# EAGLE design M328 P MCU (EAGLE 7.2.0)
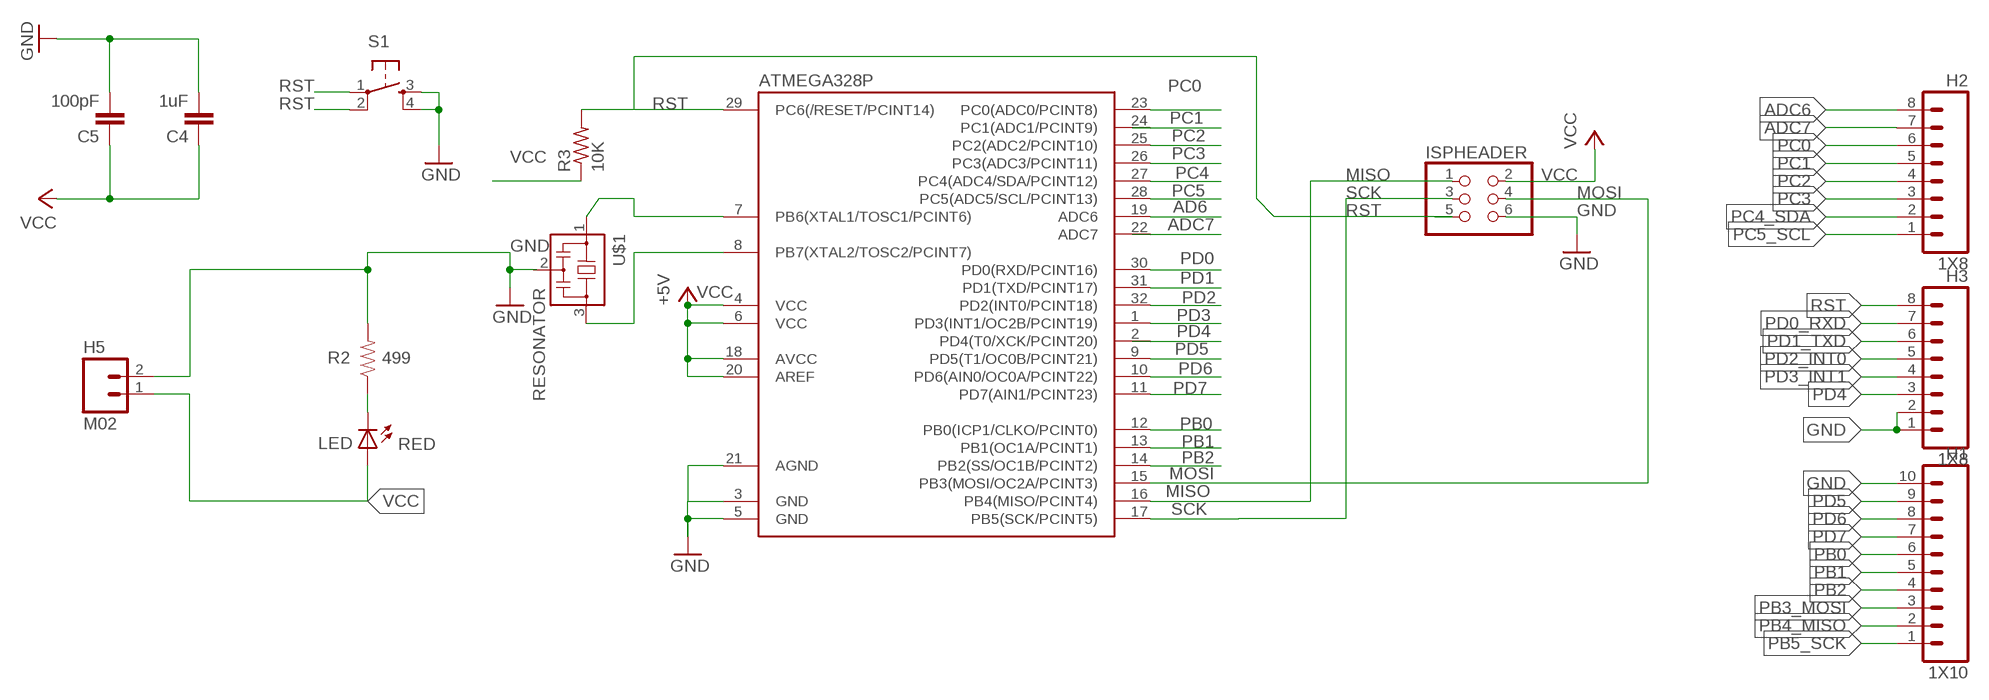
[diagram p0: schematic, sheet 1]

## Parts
ATMEGA328P  ATMEGA48/88/168-MU  [MLF32]
C4  1uF  CAP1206  [1206]
C5  100pF  CAP1206  [1206]
H1  1X10  M101X10_SMD_STRAIGHT_ALT  [1X10_SMD_STRAIGHT_ALT]
H2  1X8  M081X08_SMD_STRAIGHT_ALT  [1X08_SMD_STRAIGHT_ALT]
H3  1X8  M081X08_SMD_STRAIGHT_ALT  [1X08_SMD_STRAIGHT_ALT]
H5  M02  [1X02_SMD_FLAT_PADS]
ISPHEADER  PINHD-2X3-SMD  [2X03SMD]
LED  RED  LED1206  [1206]
R2  499  RESISTOR1206  [1206]
R3  10K  RESISTOR1206  [1206]
S1  6MM_SWITCH6MM_SWITCH  [6MM_SWITCH]
U$1  RESONATOR  [EFOBM]

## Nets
AD6: ATMEGA328P.19(ADC6)
ADC6: H2.8
ADC7: H2.7
GND: ATMEGA328P.3(GND) ATMEGA328P.5(GND) ATMEGA328P.21(AGND) C4.2 C5.2 H1.10 H3.1 H3.2 H5.2 ISPHEADER.6 R2.2 S1.3(S) S1.4(S1)
MISO: ATMEGA328P.16(PB4(MISO/PCINT4)) ISPHEADER.1
MOSI: ATMEGA328P.15(PB3(MOSI/OC2A/PCINT3)) ISPHEADER.4
N$1: ATMEGA328P.7(PB6(XTAL1/TOSC1/PCINT6)) U$1.1
N$2: ATMEGA328P.8(PB7(XTAL2/TOSC2/PCINT7)) U$1.3
N$26: LED.2(C) R2.1
PB0: ATMEGA328P.12(PB0(ICP1/CLKO/PCINT0)) H1.6
PB1: ATMEGA328P.13(PB1(OC1A/PCINT1)) H1.5
PB2: ATMEGA328P.14(PB2(SS/OC1B/PCINT2)) H1.4
PB3_MOSI: H1.3
PB4_MISO: H1.2
PB5_SCK: H1.1
PC0: ATMEGA328P.23(PC0(ADC0/PCINT8)) H2.6
PC1: H2.5
PC2: ATMEGA328P.25(PC2(ADC2/PCINT10)) H2.4
PC3: ATMEGA328P.26(PC3(ADC3/PCINT11)) H2.3
PC4: ATMEGA328P.27(PC4(ADC4/SDA/PCINT12))
PC4_SDA: H2.2
PC5: ATMEGA328P.28(PC5(ADC5/SCL/PCINT13))
PC5_SCL: H2.1
PD0: ATMEGA328P.30(PD0(RXD/PCINT16))
PD0_RXD: H3.7
PD1: ATMEGA328P.31(PD1(TXD/PCINT17))
PD1_TXD: H3.6
PD2: ATMEGA328P.32(PD2(INT0/PCINT18))
PD2_INT0: H3.5
PD3: ATMEGA328P.1(PD3(INT1/OC2B/PCINT19))
PD3_INT1: H3.4
PD4: H3.3
PD5: ATMEGA328P.9(PD5(T1/OC0B/PCINT21)) H1.9
PD6: ATMEGA328P.10(PD6(AIN0/OC0A/PCINT22)) H1.8
PD7: ATMEGA328P.11(PD7(AIN1/PCINT23)) H1.7
RST: ATMEGA328P.29(PC6(/RESET/PCINT14)) H3.8 ISPHEADER.5 R3.2 S1.1(P) S1.2(P1)
SCK: ATMEGA328P.17(PB5(SCK/PCINT5)) ISPHEADER.3
VCC: ATMEGA328P.4(VCC) ATMEGA328P.6(VCC) ATMEGA328P.18(AVCC) ATMEGA328P.20(AREF) C4.1 C5.1 H5.1 ISPHEADER.2 LED.1(A) R3.1 ; supply symbol labelled +5V
Unconnected: ATMEGA328P.2(PD4(T0/XCK/PCINT20)) ATMEGA328P.22(ADC7) ATMEGA328P.24(PC1(ADC1/PCINT9)) U$1.2

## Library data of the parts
ATMEGA328P = 01_atmega8:ATMEGA48/88/168
C4 C5 = 01_SparkFun:CAP: Capacitor
H1 = Working:M10
H2 H3 = Working:M08
H5 = Working:M02
ISPHEADER = 01_FAB_Hello:PINHD-2X3-SMD: PIN HEADER
LED = 01_FAB_Hello:LED
R2 = 01_SparkFun:RESISTOR: Resistor
R3 = 01_FAB_Hello:RESISTOR
S1 = 01_FAB_Hello:6MM_SWITCH: OMRON SWITCH
U$1 = fab-sp:RESONATOR

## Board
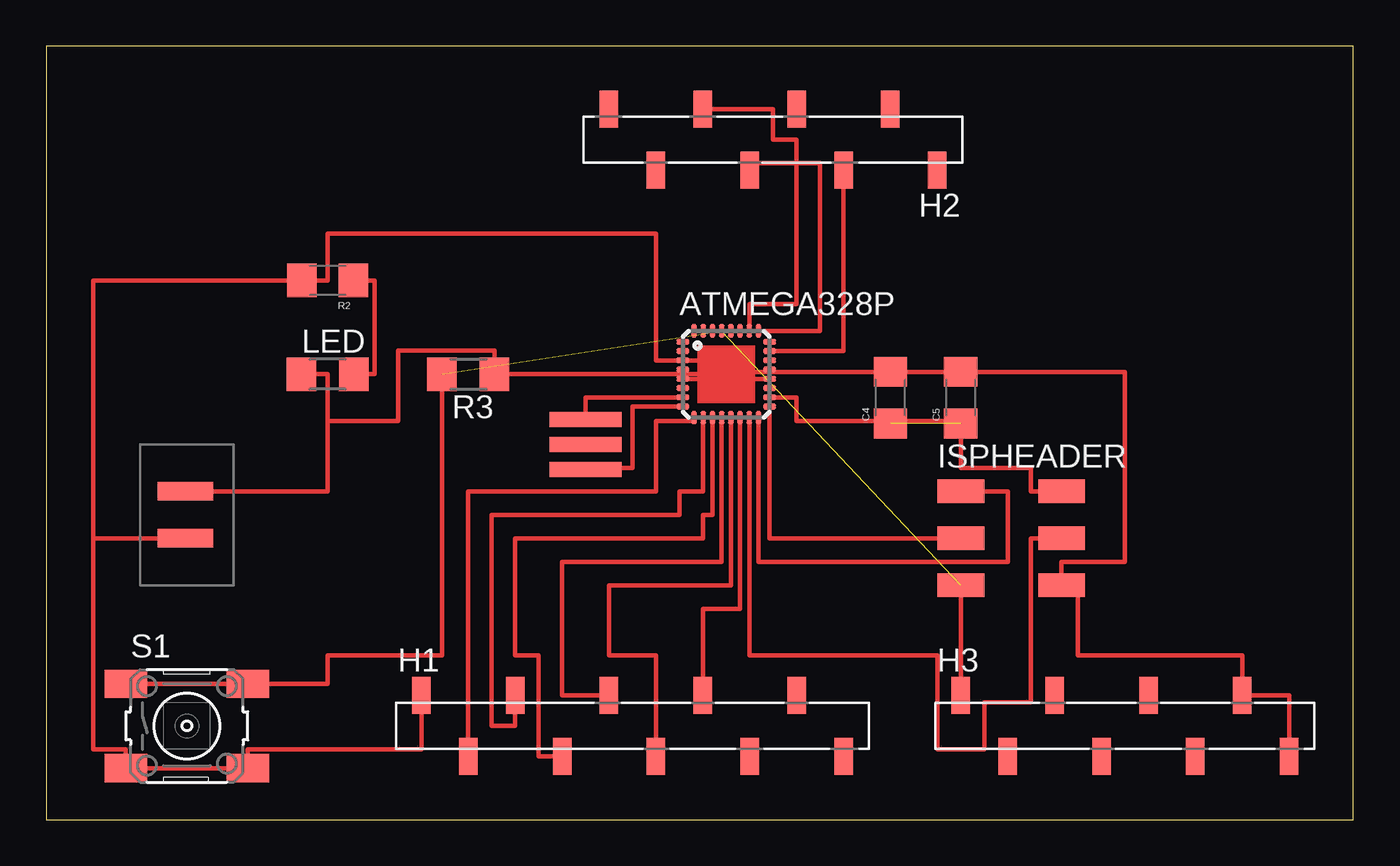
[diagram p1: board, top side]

Size 70.79 x 41.9 mm. Coordinates in mm from the lower left corner, seen from the top.
Outline: 0,0 70.79,0 70.79,41.9 0,41.9 0,0
Copper layers (1*16): Top 0.035mm / dielectric 1.5mm / Bottom 0.035mm
Design rules "default": minimum track width 10mil, minimum drill 24mil, track to track 8mil, track to pad 8mil, pad to pad 8mil, via to via 8mil, smd to smd 8mil, copper to edge 40mil, drill to drill 8mil, minimum pad ring 10mil, minimum via ring 8mil, stop-mask expansion 4mil, vias tented up to drill 0mil, thermal gap 10mil

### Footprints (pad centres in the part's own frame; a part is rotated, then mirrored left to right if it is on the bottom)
MLF32 = smd 0.7 x 0.3: 1 -2.35,1.75; 2 -2.35,1.25; 3 -2.35,0.75; 4 -2.35,0.25; 5 -2.35,-0.25; 6 -2.35,-0.75; 7 -2.35,-1.25; 8 -2.35,-1.75; 17 2.35,-1.75; 18 2.35,-1.25; 19 2.35,-0.75; 20 2.35,-0.25; 21 2.35,0.25; 22 2.35,0.75; 23 2.35,1.25; 24 2.35,1.75 | smd 0.3 x 0.7: 9 -1.75,-2.35; 10 -1.25,-2.35; 11 -0.75,-2.35; 12 -0.25,-2.35; 13 0.25,-2.35; 14 0.75,-2.35; 15 1.25,-2.35; 16 1.75,-2.35; 25 1.75,2.35; 26 1.25,2.35; 27 0.75,2.35; 28 0.25,2.35; 29 -0.25,2.35; 30 -0.75,2.35; 31 -1.25,2.35; 32 -1.75,2.35
1206 = smd 1.6 x 1.8: 1 -1.4,0; 2 1.4,0
1X10_SMD_STRAIGHT_ALT = smd 1 x 2: 1 -1.27,-0.38; 2 -3.81,2.92; 3 -6.35,-0.38; 4 -8.89,2.92; 5 -11.43,-0.38; 6 -13.97,2.92; 7 -16.51,-0.38; 8 -19.05,2.92; 9 -21.59,-0.38; 10 -24.13,2.92
1X08_SMD_STRAIGHT_ALT = smd 1 x 2: 1 -1.27,-0.38; 2 -3.81,2.92; 3 -6.35,-0.38; 4 -8.89,2.92; 5 -11.43,-0.38; 6 -13.97,2.92; 7 -16.51,-0.38; 8 -19.05,2.92
1X02_SMD_FLAT_PADS = smd 1 x 3: 1 2.54,1.19; 2 5.08,1.19
2X03SMD = smd 2.54 x 1.27: 1 -2.54,2.54; 2 2.92,2.54; 3 -2.54,0; 4 2.92,0; 5 -2.54,-2.54; 6 2.92,-2.54
1206' = smd 1.6 x 1.803: 1 -1.422,0; 2 1.422,0
6MM_SWITCH = smd 2.286 x 1.524: 1 -3.302,2.286; 2 3.302,2.286; 3 -3.302,-2.286; 4 3.302,-2.286
EFOBM = smd 0.8 x 3.9: 1 -1.35,0; 2 0,0; 3 1.35,0

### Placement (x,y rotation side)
ATMEGA328P  36.83,24.13 0 top
C4  45.72,22.86 90 top
C5  49.53,22.86 90 top
H1  44.45,3.81 0 top
H2  29.21,38.1 180 top
H3  68.58,3.81 0 top
H5  6.35,20.32 270 top
ISPHEADER  52.07,15.24 0 top
LED  RED  [1206']  15.24,24.13 0 top
R2  15.24,29.21 180 top
R3  10K  [1206']  22.86,24.13 180 top
S1  7.62,5.08 0 top
U$1  29.21,20.32 270 top

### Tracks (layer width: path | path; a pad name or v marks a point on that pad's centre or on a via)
GND
  Top 0.254: 39.18,24.26 C4.2 C5.2 58.42,24.26 58.42,13.97 54.99,13.97 ISPHEADER.6 55.88,12.7 55.88,8.89 64.77,8.89 H3.2 67.31,6.73 H3.1 | 39.18,24.26 ATMEGA328P.21 | 35.56,24.26 35.56,24.88 ATMEGA328P.3 33.02,24.88 33.02,31.75 15.24,31.75 15.24,29.21 R2.2 2.54,29.21 2.54,15.24 | ATMEGA328P.5 34.48,24.13 35.56,24.13 35.56,24.26 | H5.2 2.54,15.24 | 2.54,15.24 2.54,3.81 4.32,3.81 S1.3 S1.4 10.92,3.81 20.32,3.81 H1.10 | 39.18,24.26 35.56,24.26
MISO
  Top 0.254: ISPHEADER.1 52.07,17.78 52.07,13.97 38.58,13.97 ATMEGA328P.16
MOSI
  Top 0.254: ATMEGA328P.15 38.1,21.78 38.1,8.89 48.26,8.89 48.26,3.81 50.8,3.81 50.8,6.35 53.34,6.35 53.34,15.24 ISPHEADER.4
N$1
  Top 0.254: ATMEGA328P.7 29.21,22.88 U$1.1
N$2
  Top 0.254: ATMEGA328P.8 31.75,22.38 31.75,19.05 29.21,19.05 U$1.3
N$26
  Top 0.254: LED.2 17.78,24.13 17.78,29.21 R2.1
PB0
  Top 0.254: H1.6 27.94,6.73 27.94,13.97 36.58,13.97 ATMEGA328P.12
PB1
  Top 0.254: H1.5 33.02,8.89 30.48,8.89 30.48,12.7 37.08,12.7 ATMEGA328P.13
PB2
  Top 0.254: H1.4 35.56,11.43 37.58,11.43 ATMEGA328P.14
PC0
  Top 0.254: ATMEGA328P.23 43.18,25.38 H2.6
PC2
  Top 0.254: ATMEGA328P.25 41.91,26.48 41.91,35.56 38.1,35.56 H2.4
PC3
  Top 0.254: H2.3 39.37,38.48 39.37,36.83 40.64,36.83 40.64,27.94 38.08,27.94 ATMEGA328P.26
PD5
  Top 0.254: H1.9 22.86,17.78 33.02,17.78 33.02,21.59 35.08,21.59 ATMEGA328P.9
PD6
  Top 0.254: ATMEGA328P.10 35.56,21.78 35.56,17.78 34.29,17.78 34.29,16.51 24.13,16.51 24.13,5.08 25.4,5.08 H1.8
PD7
  Top 0.254: H1.7 26.67,3.43 26.67,8.89 25.4,8.89 25.4,15.24 35.56,15.24 35.56,16.51 36.08,16.51 ATMEGA328P.11
RST  (2 unrouted)
  Top 0.254: H3.8 ISPHEADER.5 | R3.2 21.44,8.89 15.24,8.89 15.24,7.37 S1.2 S1.1
SCK
  Top 0.254: ISPHEADER.3 39.18,15.24 ATMEGA328P.17
VCC  (1 unrouted)
  Top 0.254: ISPHEADER.2 53.34,17.78 53.34,19.05 49.53,19.05 C5.1 49.53,21.59 40.64,21.59 40.64,22.88 ATMEGA328P.18 ATMEGA328P.20 34.48,23.88 ATMEGA328P.4 | ATMEGA328P.4 ATMEGA328P.6 | ATMEGA328P.4 34.48,24.13 R3.1 24.28,25.4 19.05,25.4 19.05,21.59 15.24,21.59 | LED.1 15.24,24.13 15.24,21.59 | 15.24,21.59 15.24,17.78 H5.1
